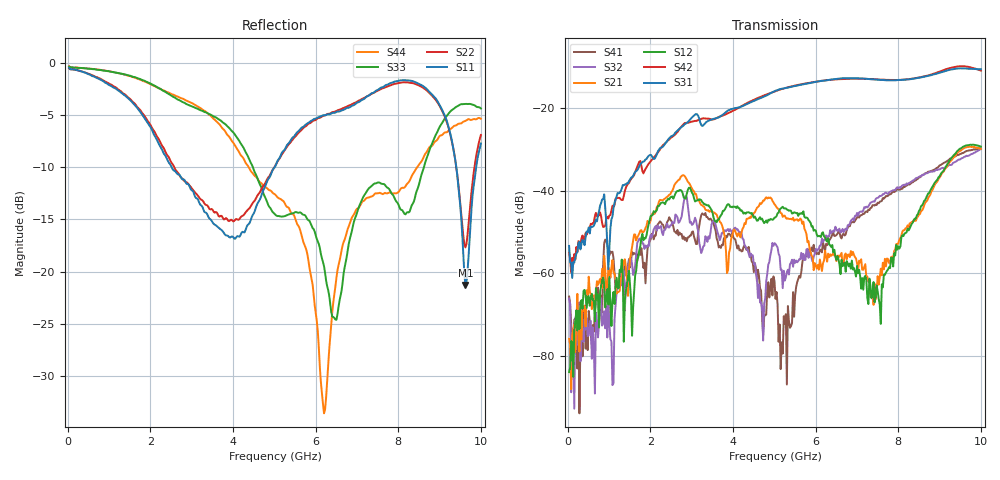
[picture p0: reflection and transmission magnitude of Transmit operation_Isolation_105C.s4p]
! Device:  ADRF5545A
! Description: Dual-Channel, Receiver Front End
! Frequency:  2.4 -  4.2 GHz
! Ports:
!	ANT-CHA	= Port 1
!	ANT-CHB	= Port 2
!  TXOUT-CHA = Port 3
!	TXOUT-CHB = Port 4
! VDD1-CHA, VDD1-CHB, VDD2-CHA, VDD2-CHB, and SWVDD-CHAB = 5 V
! SWCTRL-CHAB = 0 V,  PD-CHAB = 0 V,BP-CHA=BP-CHB=0V
! Temp=105C
! Data:  Data was collected using a calibrated 4 port network analyzer and de-embedded using AtaiTec's In Situ De-Embedding.
! Note:  Analog Devices supplies this data as a sample of measured data
!  for this product.  Your particular data for this product may vary.
!  Data was taken at 105 degrees C.
!  Analog Devices reserves the right to change this data at anytime.
!Correction: S11(Full 4 Port(1,2,3,4))
!S12(Full 4 Port(1,2,3,4))
!S13(Full 4 Port(1,2,3,4))
!S14(Full 4 Port(1,2,3,4))
!S21(Full 4 Port(1,2,3,4))
!S22(Full 4 Port(1,2,3,4))
!S23(Full 4 Port(1,2,3,4))
!S24(Full 4 Port(1,2,3,4))
!S31(Full 4 Port(1,2,3,4))
!S32(Full 4 Port(1,2,3,4))
!S33(Full 4 Port(1,2,3,4))
!S34(Full 4 Port(1,2,3,4))
!S41(Full 4 Port(1,2,3,4))
!S42(Full 4 Port(1,2,3,4))
!S43(Full 4 Port(1,2,3,4))
!S44(Full 4 Port(1,2,3,4))
!S4P File: Measurements: <S11,S12,S13,S14>,
!<S21,S22,S23,S24>,
!<S31,S32,S33,S34>,
!<S41,S42,S43,S44>:
# Hz S  dB  R 50
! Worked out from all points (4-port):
!   400 points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, 34.98 MHz to 10 GHz, reference 50 ohm
!   strongest paths, dB at 34.98 MHz, 2.532 GHz, 5.03 GHz, 7.527 GHz, 10 GHz:
!     S31: -53.3, -26.6, -15.7, -13.0, -10.5
!     S42: -55.0, -26.9, -15.8, -13.0, -10.8
!     S12: -83.9, -41.4, -46.4, -66.2, -29.2
!     S21: -75.9, -40.0, -43.5, -62.8, -29.8
!     S32: -66.1, -47.5, -52.9, -41.5, -29.8
!     S41: -65.6, -47.8, -66.2, -43.0, -29.5
!   lowest |S11| = -21.3 dB at 9.625 GHz (marker M1), VSWR 1.19, Z = 44.4 + j5.93 ohm
!   |S11| at or under -10 dB: 2.518 GHz to 5.008 GHz (2.491 GHz wide, 66.2 % of centre); 9.405 GHz to 9.887 GHz (481.7 MHz wide, 4.99 % of centre)
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3.4975e7  -0.46 -10.3  -83.93 -105.8  -51.83 -5.8  -70.72 143.5
          -75.88 152.5  -0.52 -10.1  -66.24 177.4  -54.97 -22.3
          -53.34 -13.6  -66.12 40.0  -0.34 -5.9  -67.29 -1.9
          -65.63 -157.8  -54.96 -3.4  -62.80 -14.9  -0.31 -5.8
3.331675e9  -14.33 0.4  -43.23 21.0  -23.61 79.7  -66.46 86.7
            -44.55 -3.5  -13.58 9.9  -61.25 82.7  -23.94 85.4
            -23.53 64.5  -51.00 73.4  -4.73 -137.7  -71.92 66.9
            -45.36 47.5  -22.44 67.0  -76.61 -126.5  -4.64 -127.4
5.3047e9  -7.91 52.8  -44.49 -42.5  -14.85 6.3  -58.05 68.1
          -46.77 -52.1  -8.06 57.4  -59.24 46.0  -14.79 14.3
          -14.99 7.9  -59.70 90.0  -14.59 124.7  -63.19 -176.4
          -86.97 16.3  -14.93 15.5  -68.59 145.5  -13.80 144.4
6.2038e9  -5.00 66.1  -51.04 -95.1  -13.23 -27.6  -51.82 -2.4
          -56.91 -50.7  -5.06 70.0  -54.19 -16.2  -13.18 -19.8
          -13.24 -26.9  -51.95 6.1  -19.48 127.8  -50.84 146.5
          -53.59 -5.0  -13.23 -18.7  -49.82 141.0  -33.58 -144.7
7.577425e9  -2.38 44.7  -72.26 69.0  -13.17 -74.3  -42.92 -107.4
            -58.86 4.2  -2.51 52.6  -43.93 -108.0  -13.14 -65.3
            -13.08 -74.1  -41.23 -101.7  -11.55 -82.4  -32.69 40.7
            -42.55 -110.0  -12.98 -64.9  -33.00 40.1  -12.49 -73.0
9.625375e9  -21.27 129.8  -29.03 -109.8  -10.32 -156.9  -30.61 60.3
            -29.45 -115.6  -17.68 140.9  -32.95 57.9  -9.74 -145.6
            -10.31 -157.4  -31.67 63.4  -3.93 -175.0  -31.92 -154.3
            -30.48 60.3  -9.79 -146.3  -31.98 -156.4  -5.56 -156.5
1e10  -7.72 -153.4  -29.24 -169.8  -10.48 172.8  -29.54 18.4
      -29.83 -176.0  -6.90 -161.5  -31.30 15.8  -10.71 -178.4
      -10.50 172.2  -29.83 20.3  -4.37 -161.9  -28.65 -173.8
      -29.51 15.6  -10.81 -178.9  -28.95 -177.4  -5.36 -150.4
